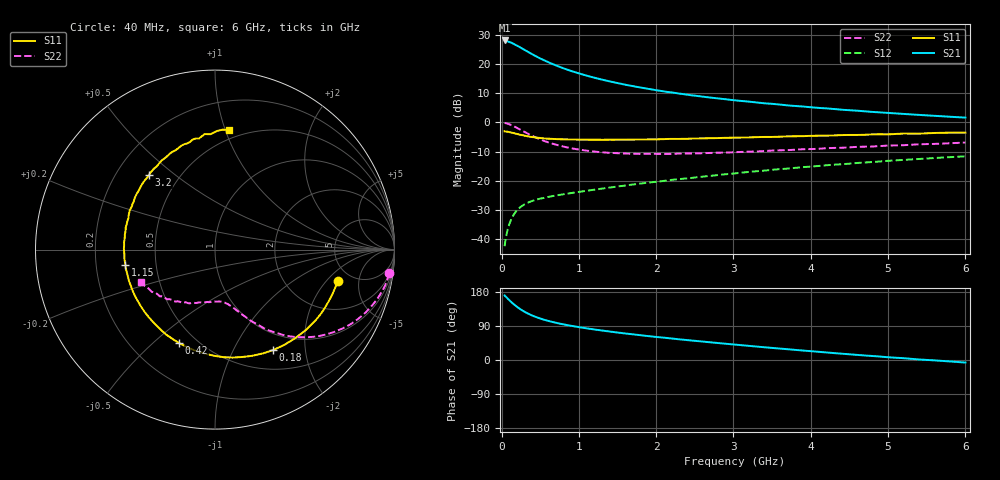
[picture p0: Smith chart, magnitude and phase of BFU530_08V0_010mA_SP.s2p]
! Filename:  P:\Prog\Test\Noise\ATS_data\Testdata_Net\03 Spar\BFU530_APG2013_40_A05_08p0V_010mA_SP_CM01_D.s2p
! Date/Time: Fri 26/Apr/2013 13:03:13
! BFU530_APG2013_40_A05_08p0V_1to25mA_SP_CM01_Bias5_R.s2p
! MDIF S-parameter v. bias file
! BFU530_APG2013_40_A05_08p0V_1to25mA_SP_CM01
! Date/time Wed Apr 24 16:58:28 2013
! VAR V_out= 8.0000
! VAR I_out= 10.0000
! VAR V_in= 0.8202
! VAR I_in= 0.1059
! Device data file deembeded for feedlines and parallel
! Original file: \03 Spar\BFU530_APG2013_40_A05_08p0V_010mA_SP_CM01_R.s2p
! Feed-files: PR047V01_250413_Feed1.s2p, PR047V01_250413_Feed2.s2p
! Parallel-file: PR047V01_250413_Par.s2p
# MHz S MA R 50
!  Freq-MHz  S11-mag  S11-arg  S21-mag  S21-arg  S12-mag  S12-arg  S22-mag  S22-arg
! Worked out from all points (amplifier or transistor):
!   98 points, 40 MHz to 6 GHz, reference 50 ohm
!   highest |S21| = 28.1 dB at 40 MHz (marker M1)
!   |S21| within 3 dB of that: start of sweep to 282 MHz
!   unconditionally stable (mu >= 1): 1.801 GHz to 3.898 GHz; 3.972 GHz to 4.003 GHz
!   at 300 MHz: K = 0.30, MSG = 26.4 dB, |S12| = -28.0 dB
!   at 1.6 GHz: K = 0.97, MSG = 17.3 dB, |S12| = -21.6 dB
!   at 6 GHz: K = 0.87, MSG = 6.6 dB, |S12| = -11.6 dB
!   S11 on the Smith chart (normalised r, x): 40 MHz: 3.85, -2.67; 180 MHz: 0.76, -1.45; 420 MHz: 0.40, -0.61; 1.15 GHz: 0.33, -0.08; 3.2 GHz: 0.34, +0.41; 6 GHz: 0.43, +1.03
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40  0.7055 -14.3  25.34 170.5  0.007632 83.3  0.9805 -7.8
50  0.7024 -17.9  25.27 167.9  0.009446 81.6  0.9752 -9.8
120  0.6757 -41.7  23.39 154.1  0.02114 70.9  0.9094 -22.7
140  0.6655 -48.1  22.74 150.3  0.02399 68.2  0.8852 -26.0
180  0.6466 -59.9  21.34 143.6  0.02913 63.4  0.8341 -31.9
220  0.6266 -70.9  20.04 137.3  0.03333 59.5  0.7823 -37.0
280  0.6019 -85.1  18 129.4  0.03839 54.8  0.7085 -43.5
340  0.5787 -97.5  16.23 122.7  0.04233 51.4  0.6441 -48.7
420  0.5577 -111.0  14.18 115.5  0.04644 48.3  0.5719 -54.0
480  0.5464 -119.5  12.89 111.0  0.04893 46.7  0.5278 -57.2
550  0.5333 -128.4  11.62 106.2  0.05116 45.5  0.4828 -60.2
650  0.524 -138.4  10.14 100.8  0.05461 44.7  0.4376 -63.8
800  0.5147 -150.2  8.471 94.1  0.05903 44.5  0.3869 -67.8
1050  0.5073 -165.6  6.619 85.1  0.0662 45.4  0.3365 -73.1
1150  0.5063 -170.3  6.078 82.0  0.06921 45.9  0.3233 -74.8
1600  0.5077 171.8  4.434 70.0  0.08325 47.7  0.2941 -82.6
2050  0.5164 159.0  3.481 59.9  0.09817 48.6  0.2894 -90.3
3100  0.5513 133.2  2.336 39.2  0.1379 47.7  0.3133 -108.7
3200  0.5547 131.7  2.274 37.3  0.1426 47.4  0.3166 -110.0
4100  0.5943 113.5  1.777 21.6  0.18 43.0  0.3543 -125.7
5200  0.6462 95.1  1.401 4.8  0.2289 35.5  0.4081 -143.7
6000  0.6702 83.4  1.211 -6.7  0.2635 28.7  0.4532 -156.2
